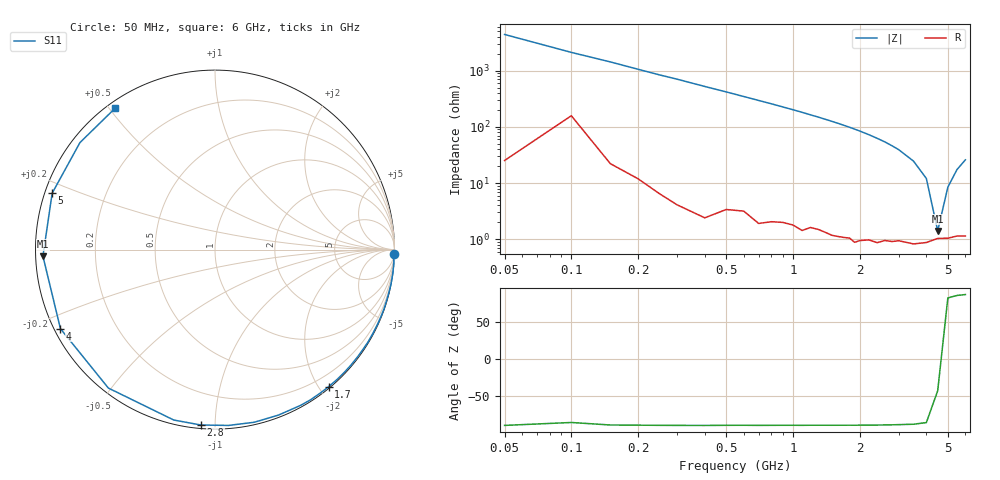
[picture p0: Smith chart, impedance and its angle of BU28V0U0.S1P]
! Infineon Technologies  Discrete & RF Semiconductors
! BB 833
! Si Tuning Diode in SOD323
! VR = 28 V
! S-Parameters:  June  1999
# GHz  S  MA  R  50
!  f  S11
! GHz  MAG  ANG
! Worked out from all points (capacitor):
!   34 points, 50 MHz to 6 GHz, reference 50 ohm
!   read as one part to ground: C = 740 fF near 50 MHz
!   lowest |Z| = 1.41 ohm at 4.5 GHz (marker M1)
!   series resonance near 4.551 GHz, so ESL is about 1.7 nH
!   S11 on the Smith chart (normalised r, x): 50 MHz: 1, -88; 1.7 GHz: 0.02, -2.13; 2.8 GHz: 0.02, -0.92; 4 GHz: 0.02, -0.24; 5 GHz: 0.02, +0.17; 6 GHz: 0.02, +0.52
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0.05  0.9999 -1.3
0.1  0.9965 -2.7
0.15  0.9989 -4.0
0.25  0.9991 -6.8
0.4  0.9991 -10.9
0.6  0.9974 -16.4
0.7  0.9979 -19.2
0.8  0.997 -22.0
1  0.9959 -27.8
1.1  0.996 -30.8
1.2  0.9945 -33.9
1.4  0.9937 -40.2
1.6  0.9929 -46.8
1.7  0.9922 -50.3
1.8  0.9914 -53.8
1.9  0.9919 -57.5
2  0.9902 -61.2
2.2  0.9875 -69.0
2.4  0.9865 -77.2
2.6  0.9826 -85.6
2.8  0.9805 -94.6
3  0.9769 -103.6
3.5  0.9737 -127.6
4  0.9674 -152.9
4.5  0.9594 -177.8
5  0.9601 160.9
5.5  0.96 141.6
6  0.9646 125.2
